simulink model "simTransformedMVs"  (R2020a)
settings: Solver=ode15s  StartTime=0.0  StopTime=tsim  MaxStep=0.01  RelTol=1e-3
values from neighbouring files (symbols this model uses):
  d1_step = 60    [runTransformedMVs.m]
  d1_step_cb = d1stepcb(n)    [runTransformedMVs.m]
  d1nom = T0nom    (= 10)    [runTransformedMVs.m]
  d2_step = d2nom*0.5    (= 0.005)    [runTransformedMVs.m]
  d2nom = qnom    (= 0.01)    [runTransformedMVs.m]
  Kc = 0    [PI_Tank.m]    (also in runCascade.m = tauQ/(tauC+theta); runTransformedMVs.m = 0.01; Main.m = 1/k*tau/(tauC+theta); runTransf.m = 1/kM(i)*tau(i)/(tauCM(i)+theta(i)))
  p = [V;rho;cp;qnom;MV;transf]    [PI_Tank.m]    (also in runCascade.m = [V;rho;cp;A;tau0;MV;transf]; runTransformedMVs.m = [V;rho;cp;A;tau0;MV;transf]; Main.m = [N, Fc0, rhoc, rhoh,U,A,cpc,cph]; Main_OL.m = [N, Fc0, rhoc, rhoh,U,A,cpc,cph])
  tauI = 1    [PI_Tank.m]    (also in runCascade.m = min(tauQ,4*(tauC+theta)); runTransformedMVs.m = 400; Main.m = min(tau,4*(tauC+theta)); runTransf.m = min(tau(i), 4*(tauCM(i)+theta(i))))
  Tnom = 50    [PI_Tank.m]    (also in runCascade.m; runTransformedMVs.m)
  transf = p(7)    [CalcBlock.m]    (also in CalcBlock_num.m; CalcBlock_v.m; PI_Tank.m = j; runCascade.m = j)
  Tstep = Tnom+10    (= 60)    [PI_Tank.m]    (also in runCascade.m = 40; runTransformedMVs.m = -10)
  tstep_d1 = 150    [runTransformedMVs.m]
  tstep_d2 = 20000    [runTransformedMVs.m]
  tstep_T1 = 100    [runTransformedMVs.m]
  tstep_T2 = 3000    [runTransformedMVs.m]
  vbias = Tnom    (= 50)    [runCascade.m]    (also in runTransformedMVs.m = 0)
  vbias_step = -A*(Tnom+Tstep)    (= 0.04)    [runTransformedMVs.m]
undefined symbols (not defined in the file or in its folder): CalcBlock, Tank

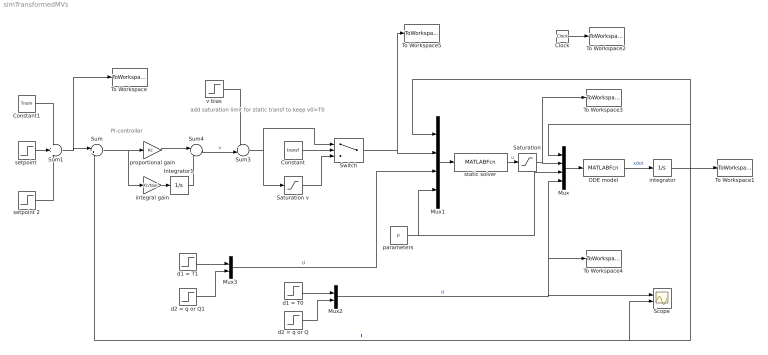
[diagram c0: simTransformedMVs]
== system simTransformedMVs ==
  note: add saturation limit for static transf to keep v0>T0
  note: PI-controller
  " integrator" : Integrator  InitialCondition=Tnom
  Clock : Clock
  Constant : Constant  Value=transf
  Constant1 : Constant  Value=Tnom
  Integrator1 : Integrator
  Mux : Mux
  Mux1 : Mux
  Mux2 : Mux  Inputs=2
  Mux3 : Mux  Inputs=2
  ODE model : MATLABFcn  MATLABFcn=Tank(u(1), u(2),u(3:9),u(10:11))  OutputDimensions=1
  Saturation : Saturate  UpperLimit=inf  LowerLimit=0
  Saturation v : Saturate  UpperLimit=inf  LowerLimit=-inf
  Scope : Scope  NumInputPorts=2
  Sum : Sum  Inputs=|+-
  Sum1 : Sum  Inputs=+++
  Sum3 : Sum  Inputs=++|
  Sum4 : Sum  Inputs=|++
  Switch : Switch  Criteria=u2 ~= 0
  To Workspace : ToWorkspace  VariableName=Tsp  SampleTime=-1
  To Workspace1 : ToWorkspace  VariableName=T  SampleTime=-1
  To Workspace2 : ToWorkspace  VariableName=time  SampleTime=-1
  To Workspace3 : ToWorkspace  VariableName=u  SampleTime=-1
  To Workspace4 : ToWorkspace  VariableName=d  SampleTime=-1
  To Workspace5 : ToWorkspace  VariableName=v  SampleTime=-1
  d1 = T0 : Step  Time=tstep_d1  Before=d1nom  After=d1_step  SampleTime=0
  d1 = T1 : Step  Time=tstep_d1  Before=d1nom  After=d1_step_cb  SampleTime=0
  d2 = q or Q : Step  Time=tstep_d2  Before=d2nom  After=d2_step  SampleTime=0
  d2 = q or Q1 : Step  Time=tstep_d2  Before=d2nom  After=d2_step  SampleTime=0
  integral gain : Gain  Gain=Kc/tauI  Multiplication=Matrix(K*u)
  parameters : Constant  Value=p
  proportional gain : Gain  Gain=Kc  Multiplication=Matrix(K*u)
  "setpoint " : Step  Time=tstep_T1  After=Tstep  SampleTime=0
  setpoint 2 : Step  Time=tstep_T2  After=-Tstep  SampleTime=0
  static solver : MATLABFcn  MATLABFcn=CalcBlock(u(1),u(2),u(3:4),u(5:11))  OutputDimensions=1
  v bias : Step  Time=tstep_T1  Before=vbias  After=vbias_step  SampleTime=0
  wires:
  " integrator"/1 -> Mux/1, Mux1/1, Scope/2, Sum/2, To Workspace1/1  "T"
  Mux/1 -> ODE model/1
  Clock/1 -> To Workspace2/1
  Sum/1 -> integral gain/1, proportional gain/1
  static solver/1 -> Saturation/1  "u"
  Sum4/1 -> Sum3/2  "v"
  Mux1/1 -> static solver/1
  ODE model/1 -> " integrator"/1  "xdot"
  integral gain/1 -> Integrator1/1
  proportional gain/1 -> Sum4/1
  Integrator1/1 -> Sum4/2
  Mux2/1 -> Scope/1, Mux/4, To Workspace4/1  "d"
  parameters/1 -> Mux/3, Mux1/4
  Sum3/1 -> Saturation v/1, Switch/1
  Saturation/1 -> Mux/2, To Workspace3/1
  Switch/1 -> Mux1/2, To Workspace5/1
  Saturation v/1 -> Switch/3
  Constant/1 -> Switch/2
  "setpoint "/1 -> Sum1/2
  Sum1/1 -> To Workspace/1, Sum/1
  setpoint 2/1 -> Sum1/3
  d1 = T0/1 -> Mux2/1
  d2 = q or Q/1 -> Mux2/2
  Constant1/1 -> Sum1/1
  d2 = q or Q1/1 -> Mux3/2
  d1 = T1/1 -> Mux3/1
  Mux3/1 -> Mux1/3  "d"
  v bias/1 -> Sum3/1
